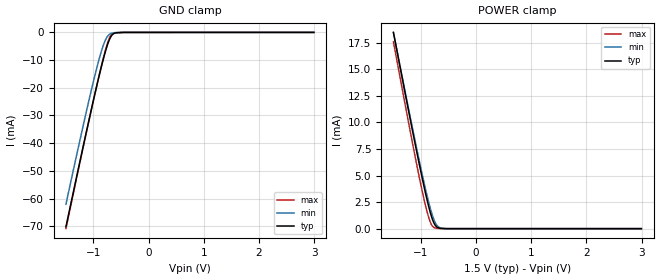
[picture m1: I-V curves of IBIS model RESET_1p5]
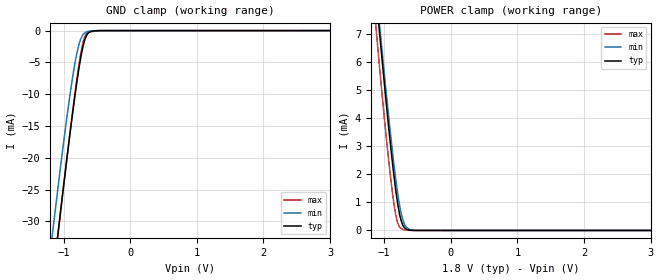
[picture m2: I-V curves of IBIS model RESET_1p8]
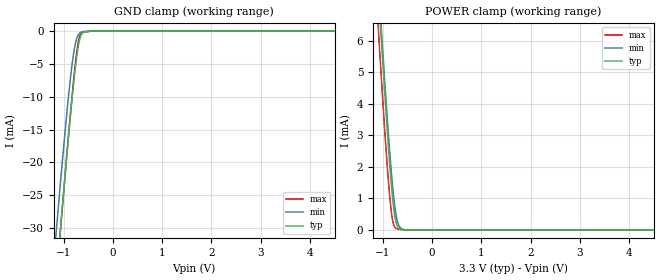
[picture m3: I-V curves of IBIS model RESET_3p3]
|Texas Instruments Incorporated
|1.2V to 3.6V, 12-Bit, Nanopower, 4-Wire
|   TOUCH SCREEN CONTROLLER with I2C Interface
| Marketing part#   Digital Voltage Range   Package-type   #pins
|TSC2004IRTJR   1.2 to 3.6   QFN   20
|TSC2004IRTJRG4   1.2 to 3.6   QFN   20
|TSC2004IRTJT   1.2 to 3.6   QFN   20
|TSC2004IRTJTG4   1.2 to 3.6   QFN   20
|TSC2004IYZKR   1.2 to 3.6   DSBGA   24
|TSC2004IYZKT   1.2 to 3.6   DSBGA   24
[IBIS Ver]   4.2
[File name]   tsc2004.ibs
[File Rev]   2.0
[Date]   03/14/2011
[Source]   Texas Instruments Incorporated.
   Analog-eLab, HPA
   12500 TI Blvd
   Dallas, TX -75243
   For Support e-mail: elab_ibis@list.ti.com
[Notes]   Revision History
   1.0: September 19, 2007
   - The following is an IBIS list for the TSC2004.
   - Please contact sllibis@ti.com with questions and
   comments concerning SLL IBIS models.
   - Data created from TI-SPICE simulations at TI-SLL.
   2.0: 03/14/2011
   - Model generated from simulations in TISPICED
   - Added DSBGA package
   - Model names with a trailing _1p5 contains the model for
   1.5V (1.2V and 1.8V).
   _ Model names with trailing _1p8 contains
   the model for 1.8V (1.65V and 2V) operation.
   _ Model names with trailing _3p3 contains
   the model for 3.3V (3V and 3.6V) operation.
   - Model not matched to measurements
   - C_comp although listed in numerical order of value are
   obtained from varying PVT conditions. For PVT conditions
   for each specific value refer the buffer description under
   respective [Model]. IBIS model user is responsible for using
   appropriate C_comp to simulate for Signal Integrity.
   3.0: 03/22/2011
   - Re-simulated I2C buffers.
[Disclaimer]
  This model is designed as an aid for customers of Texas Instruments.
  TI and its licensors and suppliers make no warranties, either expressed
  or implied, with respect to this model, including the warranties of
  merchantability or fitness for a particular purpose.  The model is
  provided solely on an "as is" basis.  The entire risk as to its quality
  and performance is with the customer.
[Copyright] (C) Copyright 2011 Texas Instruments Incorporated.
   All rights reserved.
| Components TSC2004_QFN 20-PIN and TSC2004_DSBGA 24-PIN
[Component]   tcs2004_qfn
[Manufacturer]   Texas Instruments, Inc.
[Package]   |RTJ, QFN 20-pin
|   typ   min   max
R_pkg   5.02000E-02   4.70000E-02   5.50000E-02
L_pkg   1.12020E-09   1.04300E-09   1.22700E-09
C_pkg   3.52333E-13   3.44000E-13   3.63000E-13
[Pin]   signal_name   model_name   R_pin   L_pin   C_pin
1   SDA   I2C   5.200e-02   1.167e-09   3.600e-13
2   SCL   I2C   4.700e-02   1.049e-09   3.440e-13
3   AD1   ADx   4.700e-02   1.055e-09   3.450e-13
4   PINTDAVB   PINTDAV   5.000e-02   1.119e-09   3.500e-13
5   RESETB   RESET   5.500e-02   1.227e-09   3.600e-13
6   DGND   GND   5.200e-02   1.167e-09   3.550e-13
7   IOVDD   POWER   4.900e-02   1.087e-09   3.480e-13
8   NC_0   NC   4.700e-02   1.054e-09   3.460e-13
9   AUX   TERM   4.900e-02   1.091e-09   3.490e-13
10   AGND   GND   5.300e-02   1.184e-09   3.620e-13
11   VREF   TERM   5.300e-02   1.181e-09   3.600e-13
12   SNSVDD   POWER   5.000e-02   1.108e-09   3.490e-13
13   xp   TERM   4.800e-02   1.075e-09   3.470e-13
14   yp   TERM   5.000e-02   1.107e-09   3.490e-13
15   SUBGND   GND   5.400e-02   1.200e-09   3.620e-13
16   xn   TERM   5.100e-02   1.141e-09   3.570e-13
17   yn   TERM   4.700e-02   1.043e-09   3.440e-13
18   SNSGND   GND   4.600e-02   1.025e-09   3.440e-13
19   NC_1   NC   4.900e-02   1.090e-09   3.490e-13
20   AD0   ADx   5.400e-02   1.204e-09   3.630e-13
[Component]   tcs2004_dsbga
[Manufacturer]   Texas Instruments, Inc.
[Package]   |YZK, WSCP 24-pin
|   typ   min   max
R_pkg   0.06355  0.0000   0.3780
L_pkg   0.8349nH 0.1520nH 2.8290nH
C_pkg   0.7800pF 0.2900pF 2.2810pF
[Pin]   signal_name   model_name   R_pin   L_pin   C_pin
A1  PINTDAV  PINTDAV  0.038   0.827nH   0.834pF
A2  DGND   GND   0.004   0.357nH   0.965pF
A3  IOVDD   POWER   0.006   0.365nH   0.776pF
A4  AUX   TERM   0.006   0.378nH   0.848pF
A5  AGND   GND   0.007   0.273nH   0.478pF
B1  RESET   RESET   0.007   0.287nH   0.503pF
B2  AD1   ADx   0.006   0.375nH   0.855pF
B3  NC   NC   0.007   0.380nH   0.787pF
B4  NC   NC   0.007   0.396nH   0.849pF
B5  VREF   TERM   0.211   1.751nH   0.869pF
C1  SCL   I2C   0.091   2.022nH   2.281pF
C2  NC   NC   0.006   0.351nH   0.703pF
C3  NC   NC   0.007   0.367nH   0.726pF
C4  NC   NC   0.004   0.287nH   0.662pF
C5  SNSVDD   POWER   0.011   0.366nH   0.560pF
D1  SDA   I2C   0.008   0.385nH   0.682pF
D2  NC   NC   0.000   0.152nH   0.409pF
D3  NC   NC   0.010   0.362nH   0.576pF
D4  SUBGND   GND   0.008   0.268nH   0.472pF
D5  XP   TERM   0.011   0.413nH   0.649pF
E1  AD0   ADx   0.233   2.269nH   0.882pF
E2  SNSGND   GND   0.232   2.302nH   0.828pF
E3  YN   TERM   0.090   0.865nH   0.290pF
E4  XN   TERM   0.140   1.635nH   0.727pF
E5  YP   TERM   0.378   2.829nH   0.907pF
| Model RESET
[Model Selector]   RESET
RESET_1p5   1.5 volt Vcc
RESET_1p8   1.8 volt Vcc
RESET_3p3   3.3 volt Vcc
|NOTES   Model RESET split into three Models RESET_1p5, RESET_1p8 and RESET_3p3
|   to accomodate vast voltage range of 1.2V - 3.6V
|   RESET_1p5 operates in voltage range of 1.2 - 1.5 - 1.8
|   RESET_1p8 operates in voltage range of 1.65 - 1.8 - 2
|   RESET_3p3 operates in voltage range of 3 - 3.3 - 3.6
|   The max pin frequency for Model RESET is 3.4MHz.Also the
|   voltage range and frequency is referenced with datasheet.
| Model ADx
[Model Selector]   ADx
ADx_1p5   1.5 volt Vcc
ADx_1p8   1.8 volt Vcc
ADx_3p3   3.3 volt Vcc
|NOTES   Model ADx split into three Models ADx_1p5, ADx_1p8 and ADx_3p3
|   to accomodate vast voltage range of 1.2V - 3.6V
|   ADx_1p5 operates in voltage range of 1.2 - 1.5 - 1.8
|   ADx_1p8 operates in voltage range of 1.65 - 1.8 - 2
|   ADx_3p3 operates in voltage range of 3 - 3.3 - 3.6
|   The max pin frequency for Model ADx is 3.4MHz.Also the
|   voltage range and frequency is referenced with datasheet.
| Model I2C
[Model Selector]   I2C
I2C_1p5   1.5 volt Vcc
I2C_1p8   1.8 volt Vcc
I2C_3p3   3.3 volt Vcc
|NOTES   Model I2C split into three Models I2C_1p5, I2C_1p8 and I2C_3p3
|   to accomodate vast voltage range of 1.2V - 3.6V
|   I2C_1p5 operates in voltage range of 1.2 - 1.5 - 1.8
|   I2C_1p8 operates in voltage range of 1.65 - 1.8 - 2
|   I2C_3p3 operates in voltage range of 3 - 3.3 - 3.6
|   The max pin frequency for Model I2C is 3.4MHz.Also the
|   voltage range and frequency is referenced with datasheet.
| Model PINTDAV
[Model Selector]   PINTDAV
PINTDAV_1p5   1.5 volt Vcc
PINTDAV_1p8   1.8 volt Vcc
PINTDAV_3p3   3.3 volt Vcc
|   TERM Model
[Model] TERM
Model_type Terminator
C_comp   1e-20   1e-20   1e-20
| variable   typ   min   max
[Voltage Range]   3.3V   1.2V   3.6V
[POWER Clamp Reference]  3.3V   1.2V   3.6V
[GND Clamp Reference]   0.0V   0.0V   0.0V
|Ambient Temperature Range 27   85   -40
[Temperature Range]   30   88   -40
| Models and submodels in the file (13): RESET_1p5 (Input), RESET_1p8 (Input), RESET_3p3 (Input), ADx_1p5 (Input), ADx_1p8 (Input), ADx_3p3 (Input), I2C_1p5 (I/O_open_drain), I2C_1p8 (I/O_open_drain), I2C_3p3 (I/O_open_drain), PINTDAV_1p5 (Output), PINTDAV_1p8 (Output), PINTDAV_3p3 (Output), TERM (Terminator)
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|NOTES   Model PINTDAV split into three Models PINTDAV_1p5, PINTDAV_1p8 and PINTDAV_3p3
|   to accomodate vast voltage range of 1.2V - 3.6V
|   PINTDAV_1p5 operates in voltage range of 1.2 - 1.5 - 1.8
|   PINTDAV_1p8 operates in voltage range of 1.65 - 1.8 - 2
|   PINTDAV_3p3 operates in voltage range of 3 - 3.3 - 3.6
|   The max pin frequency for Model PINTDAV is 3.4MHz.Also the
|   voltage range and frequency is referenced with datasheet.
| Model 1.5 V RESET
[Model]   RESET_1p5
Model_type  Input
Vinl = 0.3
Vinh = 1.05
|   typ   min   max
|   (nom PVT)   (Fast PVT)   (slow PVT)
C_comp   7.01584E-12   6.70009E-12   7.31273E-12
| Where   nom PVT is  Nominal Process, 3.3V, 25C
|   Fast PVT is Strong Process, 3.6V, -40C
|   Slow PVT is Weak Process, 3.0V, 85C
|C_comp - from L-C Tank method, L = 1nH, peak frequency ~ 1.9GHz
[Model Spec]   | power 1.5, 1.2, 1.8 V
Vinl   0.3   0.24   0.54
Vinh   1.05   0.84   1.26
[Voltage Range]   1.5   1.2   1.8
[Temperature Range]   30   88   -40
|Ambient Temperature Range 27   85   -40
[Power Clamp Reference]   1.5   1.2   1.8
[GND Clamp Reference]   0   0   0
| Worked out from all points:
|   GND clamp passes 1 mA (typ) near -0.67 V on its own axis
|   POWER clamp passes 1 mA (typ) near -0.80 V on its own axis
[GND Clamp]
|   Voltage   I(typ)   I(min)   I(max)
-1.5V     -70.22mA   -62.07mA   -70.87mA
-1.142V   -37.09mA   -29.72mA   -37.4mA
-985mV    -23.07mA   -16.37mA   -23.15mA
-899.3mV  -15.81mA   -9.735mA   -15.68mA
-837.6mV  -10.86mA   -5.578mA   -10.53mA
-783.4mV  -6.895mA   -2.724mA   -6.373mA
-723.3mV  -3.213mA   -917.5uA   -2.553mA
-703.2mV  -2.276mA   -574.5uA   -1.648mA
-663.9mV  -968.6uA   -258.3uA   -600.6uA
-614.2mV  -264.6uA   -96.64uA   -224.2uA
-459.5mV  -5.673uA   -7.741uA   -26.44uA
2.995V    0A         0A         0A
[POWER Clamp]
|   Voltage   I(typ)   I(min)   I(max)
-1.5V     18.46mA    18.45mA    17.57mA
-1.162V   9.417mA    9.639mA    8.251mA
-1.024V   5.897mA    6.219mA    4.663mA
-948.7mV  4.053mA    4.424mA    2.845mA
-861.7mV  2.107mA    2.515mA    1.079mA
-817.6mV  1.279mA    1.662mA    450.8uA
-798.1mV  960.6uA    1.332mA    274.4uA
-760mV    474.8uA    772.6uA    102.1uA
-715.3mV  164uA      341.6uA    32.47uA
-655.2mV  32.89uA    86.09uA    16.49uA
-510.6mV  1.334uA    1.583uA    1.306uA
2.995V    0A         0A         0A
| Model 1.8 V RESET
[Model]   RESET_1p8
Model_type  Input
Vinl = 0.54
Vinh = 1.26
|   typ   min   max
|   (nom PVT)   (Fast PVT)   (slow PVT)
C_comp   6.79329E-12   6.60819E-12   7.0808E-12
| Where   nom PVT is  Nominal Process, 3.3V, 25C
|   Fast PVT is Strong Process, 3.6V, -40C
|   Slow PVT is Weak Process, 3.0V, 85C
|C_comp - from L-C Tank method, L = 1nH, peak frequency ~ 1,9GHz
[Model Spec]   | power 1.8, 1.65. 2 V
Vinl   0.54   0.495   0.6
Vinh   1.26   1.155   1.4
[Voltage Range]   1.8   1.65   2
[Temperature Range]   30   88   -40
|Ambient Temperature Range 27   85   -40
[Power Clamp Reference]   1.8   1.65   2
[GND Clamp Reference]   0   0   0
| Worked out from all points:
|   GND clamp passes 1 mA (typ) near -0.66 V on its own axis
|   POWER clamp passes 1 mA (typ) near -0.80 V on its own axis
[GND Clamp]
|   Voltage   I(typ)   I(min)   I(max)
-1.8V     -98.57mA   -90.01mA   -99.58mA
-1.173V   -39.87mA   -32.43mA   -40.22mA
-1.14V    -36.91mA   -29.54mA   -37.22mA
-1.084V   -31.8mA    -24.65mA   -32.05mA
-1.068V   -30.35mA   -23.25mA   -30.58mA
-947.6mV  -19.85mA   -13.38mA   -19.84mA
-834.3mV  -10.61mA   -5.378mA   -10.27mA
-741mV    -4.194mA   -1.301mA   -3.536mA
-678.8mV  -1.353mA   -336.9uA   -923.8uA
-622mV    -324.1uA   -113.1uA   -256.7uA
-461.7mV  -6.01uA    -7.919uA   -26.67uA
3.595V    0A         0A         0A
[POWER Clamp]
|   Voltage   I(typ)   I(min)   I(max)
-1.8V     26.66mA    26.45mA    26.02mA
-1.123V   8.404mA    8.654mA    7.217mA
-1.091V   7.575mA    7.848mA    6.36mA
-1.057V   6.716mA    7.016mA    5.495mA
-949.7mV  4.075mA    4.444mA    2.866mA
-876.7mV  2.426mA    2.822mA    1.345mA
-804.4mV  1.059mA    1.429mA    323.7uA
-748.8mV  372.2uA    639.9uA    73.92uA
-694.4mV  96.96uA    215uA      27.5uA
-660.8mV  39.34uA    98.7uA     18.71uA
-511.6mV  1.446uA    1.627uA    1.242uA
3.595V    0A         0A         0A
| Model 3.3 V RESET
[Model]   RESET_3p3
Model_type  Input
Vinl = 0.99
Vinh = 2.31
|   typ   min   max
|   (nom PVT)   (Fast PVT)   (slow PVT)
C_comp   6.05456E-12   5.91615E-12   6.33989E-12
| Where   nom PVT is  Nominal Process, 3.3V, 25C
|   Fast PVT is Strong Process, 3.6V, -40C
|   Slow PVT is Weak Process, 3.0V, 85C
|C_comp - from L-C Tank method, L = 1nH, peak frequency ~ 2GHz
[Model Spec]   | power 3.3. 3, 3.6 V
Vinl   0.99   0.9   1.08
Vinh   2.31   2.1   2.52
[Voltage Range]   3.3   3   3.6
[Temperature Range]   30   88   -40
|Ambient Temperature Range 27   85   -40
[Power Clamp Reference]   3.3   3   3.6
[GND Clamp Reference]   0   0   0
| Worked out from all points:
|   GND clamp passes 1 mA (typ) near -0.67 V on its own axis
|   POWER clamp passes 1 mA (typ) near -0.80 V on its own axis
[GND Clamp]
|   Voltage   I(typ)   I(min)   I(max)
-3.3V     -242.5mA   -232.6mA   -245.1mA
-1.157V   -38.42mA   -30.99mA   -38.75mA
-1.126V   -35.61mA   -28.3mA    -35.88mA
-1.065V   -30.13mA   -23.03mA   -30.36mA
-915.1mV  -17.13mA   -10.9mA    -17.04mA
-814.2mV  -9.106mA   -4.227mA   -8.707mA
-768.1mV  -5.875mA   -2.111mA   -5.279mA
-713.3mV  -2.752mA   -740.5uA   -2.074mA
-653.8mV  -740.5uA   -196.7uA   -493.3uA
-597.1mV  -170.6uA   -61.61uA   -174uA
-453mV    -4.685uA   -7.191uA   -24.57uA
6.59V     0A         0A         0A
[POWER Clamp]
|   Voltage   I(typ)   I(min)   I(max)
-3.3V     68.31mA    67.22mA    68.84mA
-1.125V   8.457mA    8.704mA    7.272mA
-1.074V   7.156mA    7.441mA    5.929mA
-1.042V   6.329mA    6.639mA    5.105mA
-1.028V   5.995mA    6.309mA    4.764mA
-945.9mV  3.993mA    4.36mA     2.781mA
-856.7mV  2.012mA    2.418mA    995.2uA
-795.5mV  932.3uA    1.286mA    255.8uA
-728.8mV  231.2uA    442.5uA    44.82uA
-638.2mV  37.35uA    56.55uA    16.14uA
-507.5mV  1.188uA    1.405uA    1.089uA
6.59V     0A         0A         0A
